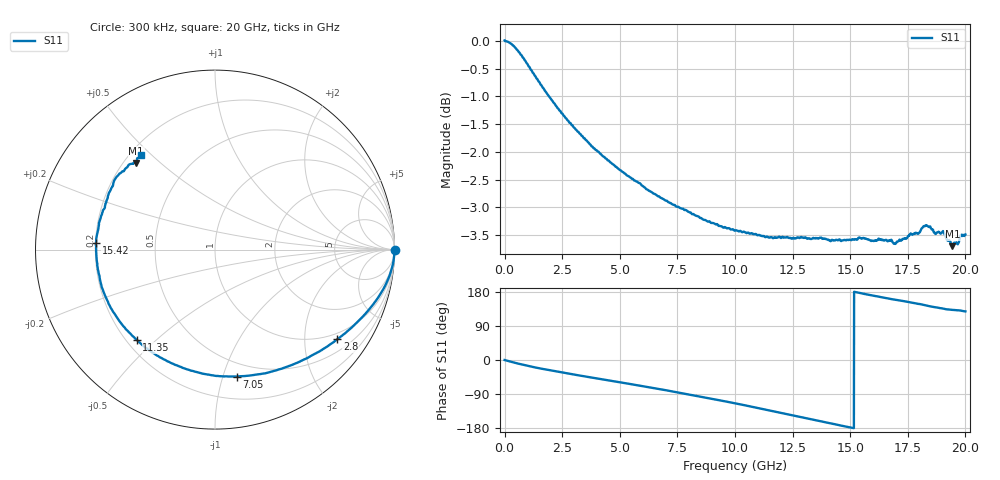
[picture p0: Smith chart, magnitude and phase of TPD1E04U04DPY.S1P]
!  1-Port S-parameters saved by WinCal
! VAR MeasName=S-Parameters (CALIBRATED_DATA) read from VNA (N5230A)
! VAR MeasDate=4/8/2016 10:06:24 AM
! VAR NAME=TPD1E04U04DPY
! VAR FILENAME=TPD1E04U04DPY.S1P
! VAR DATE=4/8/2016 10:06:24 AM
! VAR PHYS_PORTS=1
! VAR ObjTypeName=DATASET
! VAR IndexType=Frequency
! Port data:
!!!Port 1: Pin 1_In
# Hz S MA R 50
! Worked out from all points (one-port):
!   2001 points, 300 kHz to 20 GHz, reference 50 ohm
!   lowest |S11| = -3.7 dB at 19.44 GHz (marker M1), VSWR 4.76, Z = 12.4 + j20.9 ohm
!   |S11| at or under -10 dB: nowhere
!   S11 on the Smith chart (normalised r, x): 300 kHz: open; 2.8 GHz: 0.82, -2.85; 7.05 GHz: 0.38, -1.11; 11.35 GHz: 0.24, -0.43; 15.42 GHz: 0.20, +0.03; 20 GHz: 0.24, +0.46
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300000  1.001 -0.1
4.802928e8  0.9855 -7.8
1.130283e9  0.9424 -17.2
1.740274e9  0.9023 -24.6
2.500262e9  0.8603 -33.0
2.800258e9  0.8447 -36.2
3.650245e9  0.8094 -45.0
5.000225e9  0.765 -58.8
5.930211e9  0.7419 -68.5
7.050194e9  0.7175 -80.3
7.500188e9  0.7089 -85.3
8.00018e9  0.7011 -91.0
8.800168e9  0.6876 -100.2
1.000015e10  0.6744 -114.2
1.066014e10  0.6703 -122.3
1.135013e10  0.6656 -131.0
1.250011e10  0.6641 -145.8
1.298011e10  0.6644 -152.1
1.377009e10  0.6637 -162.3
1.500008e10  0.6618 -178.0
1.542007e10  0.6646 176.7
1.633006e10  0.6621 166.0
1.750004e10  0.6662 153.7
1.818003e10  0.6803 145.6
1.851002e10  0.6775 141.1
1.910001e10  0.6698 134.5
1.944001e10  0.6531 132.3
2e10  0.6692 128.3
